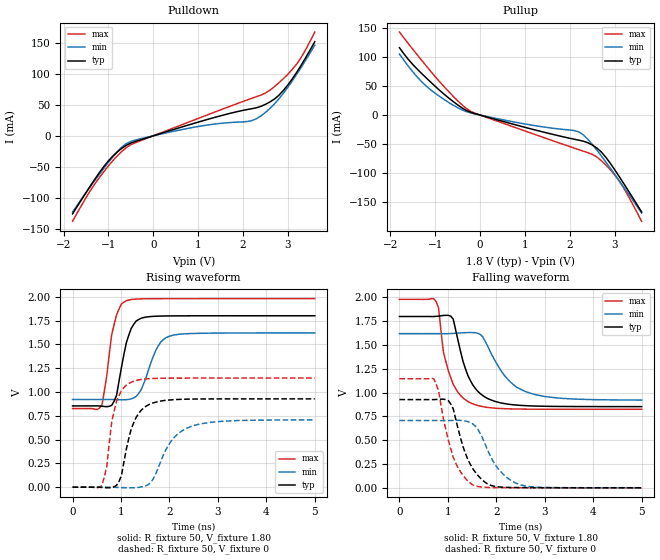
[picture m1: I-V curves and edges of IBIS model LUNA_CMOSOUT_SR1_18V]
[IBIS Ver]   3.2
[Comment Char]   |_char
[File name]   sg8201cga_18v_d.ibs
[File Rev]   1.1
[Date]   2021/10/19 9:35:58
[Source]
[Notes]
[Disclaimer]
This information is for modeling purposes only, and is not guaranteed.
Property of SEIKO EPSON Corp.,
unauthorized reproduction and/or distribution is strictly prohibited.
[Copyright]
Copyright 2021, SEIKO EPSON Corp.
[Component]   2G005_2016
Si_location Pin
Timing_location Pin
[Manufacturer]   SEIKO EPSON Corp.
| 2016 PKG
[Package]
R_pkg   42m   NA   NA
L_pkg   0.49n   NA   NA
C_pkg   0.178p   NA   NA
[Pin] signal_name   model_name
1   OE   NC
2   GND   GND
3   OUT   LUNA_CMOSOUT_SR1_18V
4   VCC   POWER
| Models and submodels in the file (1): LUNA_CMOSOUT_SR1_18V (Output)
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[Model]   LUNA_CMOSOUT_SR1_18V
Model_type Output
Polarity Non-Inverting
Vmeas=0.90
C_comp   2.5p   2.0p   3.0p
[Temperature Range] 25   140   -40
[Voltage Range]   1.80   1.62   1.98
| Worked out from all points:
|   slope of the pulldown table from 0 to 0.27 V, typ, clamps not added: 44.4 ohm
|   slope of the pullup table from 0 to 0.27 V, typ, clamps not added: 46.3 ohm
|   falling waveform, R_fixture 50, V_fixture 1.80: 20-80 % time 388ps typ, 583ps min, 309ps max; typ from 1.8 V to 0.853 V
|   falling waveform, R_fixture 50, V_fixture 0: 20-80 % time 384ps typ, 472ps min, 350ps max; typ from 0.927 V to 0.001 V
|   rising waveform, R_fixture 50, V_fixture 1.80: 20-80 % time 236ps typ, 319ps min, 207ps max; typ from 0.853 V to 1.8 V
|   rising waveform, R_fixture 50, V_fixture 0: 20-80 % time 292ps typ, 469ps min, 210ps max; typ from 0 V to 0.927 V
[Pullup]
-1.8V     116.4mA    105.5mA    143.6mA
-1.5V     87.28mA    74.66mA    113.7mA
-1.2V     64.08mA    49.96mA    84.8mA
-700mV    29.47mA    21.72mA    40.49mA
-300mV    7.706mA    5.743mA    10.92mA
900mV     -19.11mA   -13.96mA   -24.72mA
2.2V      -43.37mA   -29.11mA   -59.76mA
2.4V      -47.78mA   -41.81mA   -64.95mA
2.6V      -56.85mA   -60.41mA   -72.43mA
2.9V      -83.24mA   -91.61mA   -94.4mA
3.2V      -118.2mA   -124.4mA   -126.1mA
3.6V      -167.6mA   -169.3mA   -183.5mA
[Pulldown]
-1.8V     -125.9mA   -122.9mA   -137.8mA
-1.4V     -80.46mA   -81.57mA   -88.07mA
-1.1V     -49.28mA   -52.2mA    -57.66mA
-900mV    -32.58mA   -33.87mA   -39.88mA
-600mV    -15.21mA   -12.54mA   -18.89mA
900mV     19.93mA    13.71mA    25.18mA
2.2V      43.74mA    24.56mA    60.59mA
2.4V      47.53mA    32.04mA    65.7mA
2.8V      65.37mA    59.53mA    85.51mA
3.1V      91.9mA     88.67mA    107.1mA
3.3V      114.2mA    110.7mA    126.8mA
3.6V      151.7mA    146.1mA    167.3mA
[Falling Waveform]
R_fixture=50
V_fixture=1.80
V_fixture_min=1.62
V_fixture_max=1.98
0s        1.8V       1.62V      1.98V
757.6ps   1.801V     1.62V      1.956V
909.1ps   1.811V     1.62V      1.423V
1.01ns    1.812V     1.62V      1.23V
1.111ns   1.771V     1.622V     1.087V
1.465ns   1.127V     1.631V     893.8mV
1.818ns   939mV      1.492V     844.9mV
2.222ns   881.1mV    1.148V     830.7mV
2.626ns   862.8mV    1.007V     826.8mV
5ns       853.5mV    922mV      825.4mV
[Falling Waveform]
R_fixture=50
V_fixture=0
V_fixture_min=0
V_fixture_max=0
0s        927.4mV    707mV      1.146V
707.1ps   927mV      706.8mV    1.146V
808.1ps   930.1mV    706.7mV    1.018V
909.1ps   931.4mV    706.6mV    720.9mV
1.061ns   880.2mV    707.8mV    407mV
1.212ns   618mV      709.6mV    207.9mV
1.515ns   200.5mV    671.4mV    30.51mV
2.02ns    11.67mV    212.4mV    2.629mV
2.424ns   3.08mV     45.34mV    1.431mV
5ns       542.9uV    994.8uV    316.4uV
[Rising Waveform]
R_fixture=50
V_fixture=1.80
V_fixture_min=1.62
V_fixture_max=1.98
0s        853.4mV    920.9mV    825.4mV
606.1ps   850.4mV    921.2mV    860.5mV
707.1ps   845.4mV    921.5mV    1.172V
808.1ps   859.9mV    920.8mV    1.603V
909.1ps   966.5mV    918.8mV    1.81V
1.111ns   1.518V     919.1mV    1.959V
1.364ns   1.76V      983.7mV    1.976V
1.768ns   1.796V     1.483V     1.979V
2.02ns    1.798V     1.589V     1.98V
5ns       1.8V       1.62V      1.98V
[Rising Waveform]
R_fixture=50
V_fixture=0
V_fixture_min=0
V_fixture_max=0
0s        16.9nV     465nV      16.02nV
606.1ps   -2.337mV   169.8uV    18.13mV
707.1ps   -6.349mV   437.7uV    220.3mV
909.1ps   19.75mV    -1.82mV    905.1mV
1.01ns    123.6mV    -3.882mV   1.015V
1.212ns   614.3mV    -6.55mV    1.103V
1.566ns   864.4mV    28.27mV    1.139V
2.02ns    916.4mV    473.5mV    1.145V
2.424ns   924.9mV    633.4mV    1.146V
5ns       927.4mV    706.6mV    1.146V
[Ramp]
R_load=50
dV/dt_r   5.564E-1/2.918E-10   4.240E-1/4.665E-10   6.875E-1/2.103E-10
dV/dt_f   5.679E-1/3.877E-10   4.188E-1/5.800E-10   6.927E-1/3.086E-10
|[End   LUNA_CMOSOUT_SR1_18V
